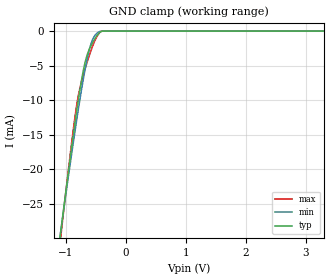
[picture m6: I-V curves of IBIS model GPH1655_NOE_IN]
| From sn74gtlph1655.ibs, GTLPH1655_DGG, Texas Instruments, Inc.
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[Model]   GPH1655_NOE_IN
Model_type  Input
Vinl=0.8
Vinh=2.0
| variable   typ   min   max
C_comp   3.67pF   2.68pF   4.40pF
[Temperature Range]   40   100   -40
| Ambient temperature   25   85   -40
[Voltage range]   3.3   3.15   3.45
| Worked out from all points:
|   GND clamp passes 1 mA (typ) near -0.51 V on its own axis
[GND Clamp]
| GPH1655_NOE_IN
|   Voltage   I(typ)   I(min)   I(max)
-5.5V     -365.8mA   -335.7mA   -411.9mA
-1.115V   -31.06mA   -30.84mA   -32.13mA
-1.075V   -28.31mA   -28.31mA   -29.01mA
-875mV    -15.03mA   -16.12mA   -14.22mA
-825mV    -11.95mA   -13.22mA   -11.07mA
-785mV    -9.613mA   -10.98mA   -9.047mA
-690mV    -4.94mA    -6.071mA   -5.796mA
-650mV    -3.605mA   -4.276mA   -4.639mA
-600mV    -2.466mA   -2.423mA   -3.302mA
-520mV    -1.158mA   -688.8uA   -1.485mA
-425mV    -126.6uA   -44.81uA   -131uA
3.3V      199.8pA    681.8pA    1.464nA
